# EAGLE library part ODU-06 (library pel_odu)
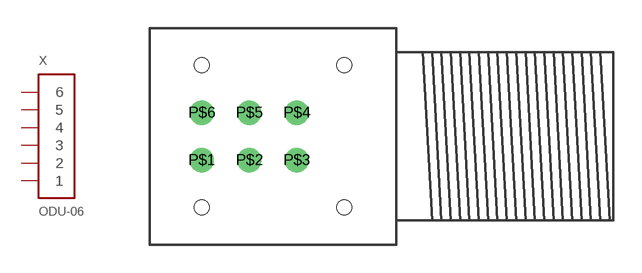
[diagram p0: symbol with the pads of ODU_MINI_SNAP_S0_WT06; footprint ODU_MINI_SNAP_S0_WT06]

Designator prefix X

## ODU-06-S0WT  [ODU_MINI_SNAP_S0_WT06]
P$1  1
P$2  2
P$3  3
P$4  4
P$5  5
P$6  6

## Footprint ODU_MINI_SNAP_S0_WT06 (pad centres in mm)
drill 0.8: P$1 -3.81,-1.27; P$2 -1.27,-1.27; P$3 1.27,-1.27; P$4 1.27,1.27; P$5 -1.27,1.27; P$6 -3.81,1.27
hole 0.8 at -3.81,3.81
hole 0.8 at 3.81,3.81
hole 0.8 at 3.81,-3.81
hole 0.8 at -3.81,-3.81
